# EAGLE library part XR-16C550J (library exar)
UART/FIFO
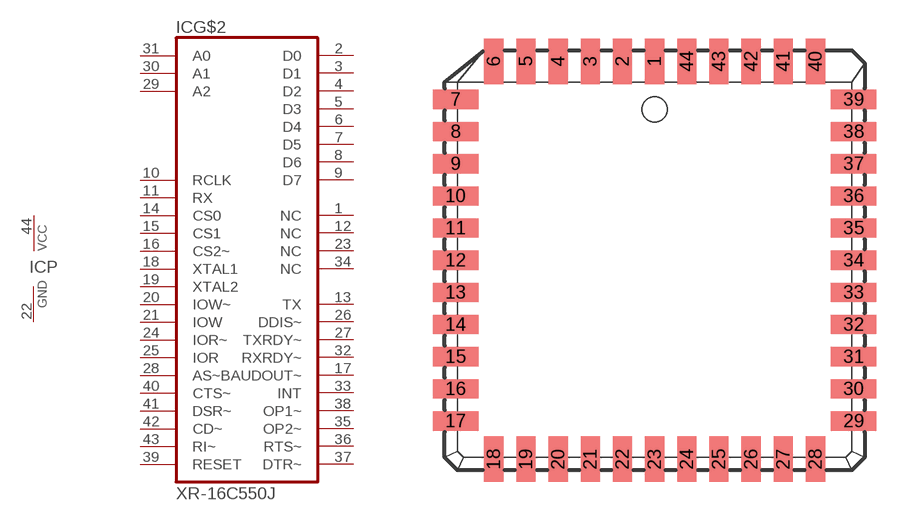
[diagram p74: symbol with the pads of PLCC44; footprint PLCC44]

Designator prefix IC; gates P=PWRN G$2=16C550J

## XR-16C550J (MPN: SC16C550BIA44; OC_FARNELL: 1564955; OC_NEWARK: 24M7289)  [PLCC44]
1  G$2:NC  nc
2  G$2:D0
3  G$2:D1
4  G$2:D2
5  G$2:D3
6  G$2:D4
7  G$2:D5
8  G$2:D6
9  G$2:D7
10  G$2:RCLK  in
11  G$2:RX  in
12  G$2:NC  nc
13  G$2:TX  out
14  G$2:CS0  in
15  G$2:CS1  in
16  G$2:CS2~  in
17  G$2:BAUDOUT~  out
18  G$2:XTAL1  in
19  G$2:XTAL2  in
20  G$2:IOW~  in
21  G$2:IOW  in
22  P:GND  pwr
23  G$2:NC  nc
24  G$2:IOR~  in
25  G$2:IOR  in
26  G$2:DDIS~  out
27  G$2:TXRDY~  out
28  G$2:AS~  in
29  G$2:A2  in
30  G$2:A1  in
31  G$2:A0  in
32  G$2:RXRDY~  out
33  G$2:INT  out
34  G$2:NC  nc
35  G$2:OP2~  out
36  G$2:RTS~  out
37  G$2:DTR~  out
38  G$2:OP1~  out
39  G$2:RESET  in
40  G$2:CTS~  in
41  G$2:DSR~  in
42  G$2:CD~  in
43  G$2:RI~  in
44  P:VCC  pwr

## Footprint PLCC44 (pad centres in mm)
Plastic Leaded Chip Carrier
smd 0.76 x 1.8: 1 0,7.86; 2 -1.27,7.86; 3 -2.54,7.86; 4 -3.81,7.86; 5 -5.08,7.86; 6 -6.35,7.86; 18 -6.35,-7.86; 19 -5.08,-7.86; 20 -3.81,-7.86; 21 -2.54,-7.86; 22 -1.27,-7.86; 23 0,-7.86; 24 1.27,-7.86; 25 2.54,-7.86; 26 3.81,-7.86; 27 5.08,-7.86; 28 6.35,-7.86; 40 6.35,7.86; 41 5.08,7.86; 42 3.81,7.86; 43 2.54,7.86; 44 1.27,7.86
smd 1.8 x 0.76: 7 -7.86,6.35; 8 -7.86,5.08; 9 -7.86,3.81; 10 -7.86,2.54; 11 -7.86,1.27; 12 -7.86,0; 13 -7.86,-1.27; 14 -7.86,-2.54; 15 -7.86,-3.81; 16 -7.86,-5.08; 17 -7.86,-6.35; 29 7.86,-6.35; 30 7.86,-5.08; 31 7.86,-3.81; 32 7.86,-2.54; 33 7.86,-1.27; 34 7.86,0; 35 7.86,1.27; 36 7.86,2.54; 37 7.86,3.81; 38 7.86,5.08; 39 7.86,6.35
